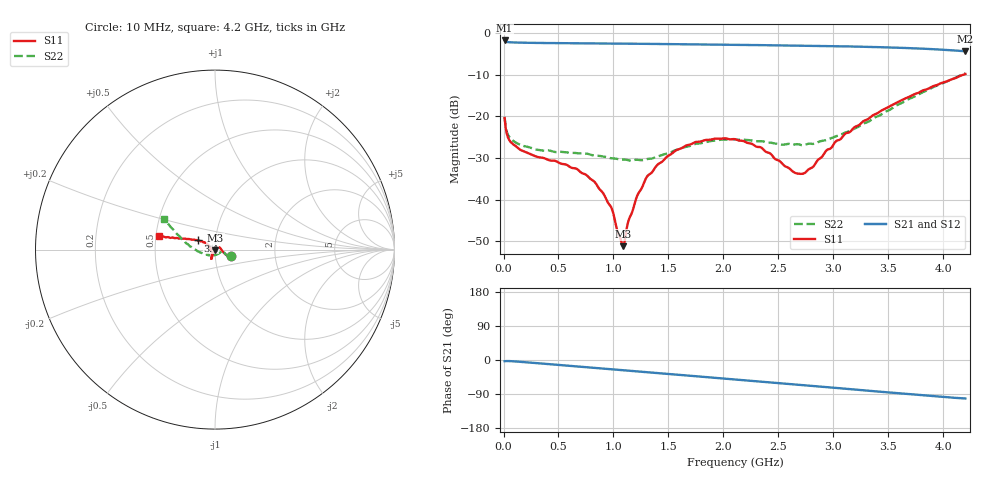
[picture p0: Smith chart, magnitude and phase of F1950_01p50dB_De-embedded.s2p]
! Integrated Device Technology
! Corporate Headquarters
! 6024 Silver Creek Valley Road
! San Jose, CA 95138  USA
! Phone:  1-408-284-8200
! Toll Free:  1-800-223-1366
! Webpage:  http://www.idt.com/
! Timing and RF Division
! 515 Groton Road, Suite 102
! Westford, MA 01886-6024
! Device:  F1950
! Description: 7-bit 0.25 dB Digital Step Attenuator
! Frequency:  150.0 -  4000.00 MHz
! Package:  4x4 mm Thin QFN Plastic Package: 24 pin
! Ports:  2 RF, 12 DC
!  Pin  1  = D0
!  Pin  2  = VDD
!  Pin  3  = Vmode
!  Pin  4  = GND
!  Pin  5  = RF1  =  Port 1
!  Pin  6  = GND
!  Pin  7  = GND
!  Pin  8  = GND
!  Pin  9  = GND
!  Pin 10  = GND
!  Pin 11  = GND
!  Pin 12  = GND
!  Pin 13  = GND
!  Pin 14  = RF2  =  Port 2
!  Pin 15  = GND
!  Pin 16  = LE
!  Pin 17  = CLK
!  Pin 18  = DATE
!  Pin 19  = D6
!  Pin 20  = D5
!  Pin 21  = D4
!  Pin 22  = D3
!  Pin 23  = D2
!  Pin 24  = D1
! State:  6
! Atten State:  1.50 dB
! Voltage:  +5.00 Volts
! Current:  Not Measured mA
! Data:  The device was measured on a the F195X evaluation board which has
!  individual transmission lines to the RF pins.  Data was collected
!  using a calibrated network analyzer.  The evaluation board was
!  de-embedded using a TRL calibration technique.
!  The reference plane is the edge of the package pin.
! Misc:  Board 2019
!  Action Tracker AT0250
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# GHz S dB R 50
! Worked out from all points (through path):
!   420 points, 10 MHz to 4.2 GHz, reference 50 ohm
!   highest |S21| = -1.77 dB at 10 MHz (marker M1); lowest = -4.4 dB at 4.2 GHz (marker M2)
!   group delay of S21, straight-line fit = 67 ps
!   lowest |S11| = -51.2 dB at 1.09 GHz (marker M3), VSWR 1.01, Z = 50.2 - j0.216 ohm
!   |S11| at or under -10 dB: start of sweep to 4.183 GHz
!   |S22| runs from -30.7 to -9.7 dB; largest |S21 - S12| = 0.00095
!   S11 on the Smith chart (normalised r, x): 10 MHz: 1.19, -0.09; 3.4 GHz: 0.82, +0.08; 4.2 GHz: 0.52, +0.09
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0.01  -20.40 -22.5  -1.77 -3.1  -1.77 -3.1  -20.23 -22.0
0.06  -26.01 -17.9  -2.21 -2.9  -2.21 -2.9  -25.20 -19.0
0.15  -27.99 -8.4  -2.30 -4.7  -2.30 -4.7  -26.79 -13.2
0.71  -33.59 37.2  -2.46 -18.0  -2.46 -18.0  -28.95 -17.2
0.82  -35.56 39.1  -2.48 -20.6  -2.48 -20.6  -29.38 -23.6
0.91  -38.62 40.3  -2.50 -22.8  -2.50 -22.8  -29.68 -31.2
0.98  -41.89 32.5  -2.52 -24.4  -2.52 -24.4  -30.08 -38.8
1.06  -49.05 -11.6  -2.54 -26.3  -2.54 -26.3  -30.38 -49.6
1.09  -51.20 -51.4  -2.55 -27.0  -2.54 -27.0  -30.40 -53.6
1.14  -44.79 -86.7  -2.56 -28.2  -2.55 -28.2  -30.59 -60.8
1.22  -38.83 -104.6  -2.57 -30.1  -2.57 -30.1  -30.45 -72.9
1.3  -34.68 -110.1  -2.59 -32.1  -2.59 -32.1  -30.32 -86.1
1.41  -31.42 -111.3  -2.62 -34.7  -2.62 -34.7  -29.58 -102.3
1.74  -26.23 -112.4  -2.71 -42.6  -2.71 -42.6  -26.67 -134.6
2.11  -25.53 -112.3  -2.82 -51.5  -2.82 -51.5  -25.57 -149.2
2.34  -27.46 -116.9  -2.90 -57.0  -2.90 -57.0  -25.97 -150.6
2.66  -33.67 -157.7  -3.00 -64.7  -3.00 -64.7  -26.72 -146.4
2.81  -32.26 163.8  -3.06 -68.4  -3.06 -68.4  -26.63 -146.4
3.03  -25.86 146.4  -3.15 -73.8  -3.15 -73.9  -24.75 -153.0
3.4  -19.26 152.2  -3.37 -83.1  -3.37 -83.2  -20.03 -175.7
3.51  -17.62 155.0  -3.45 -85.9  -3.45 -85.9  -18.47 177.4
4.2  -9.84 166.3  -4.38 -101.5  -4.37 -101.6  -9.66 148.9
